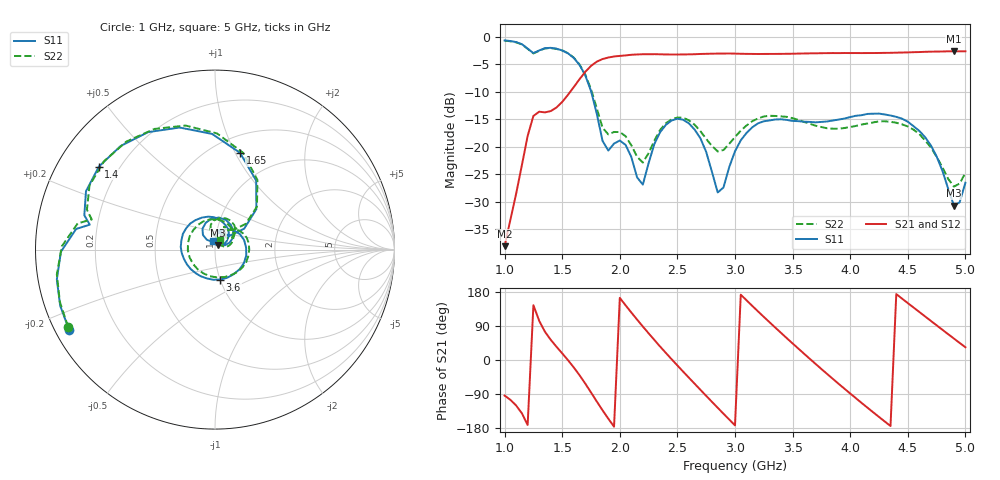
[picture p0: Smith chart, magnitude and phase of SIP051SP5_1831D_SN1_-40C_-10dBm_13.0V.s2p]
# GHz  S  dB  R  50
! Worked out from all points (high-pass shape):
!   81 points, 1 GHz to 5 GHz, reference 50 ohm
!   highest |S21| = -2.62 dB at 4.9 GHz (marker M1); lowest = -38.1 dB at 1 GHz (marker M2)
!   |S21| within 3 dB of the highest: 1.735 GHz to end of sweep
!   lowest |S11| = -30.7 dB at 4.9 GHz (marker M3), VSWR 1.06, Z = 51.7 + j2.44 ohm
!   |S11| at or under -10 dB: 1.752 GHz to end of sweep
!   |S22| runs from -27.2 to -0.7 dB; largest |S21 - S12| = 0.0023
!   S11 on the Smith chart (normalised r, x): 1 GHz: 0.04, -0.26; 1.4 GHz: 0.13, +0.32; 1.65 GHz: 0.67, +1.05; 3.6 GHz: 1.00, -0.34; 5 GHz: 0.97, +0.09
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1  -0.65 -151.2  -38.09 -93.9  -37.92 -92.7  -0.68 -152.2
1.25  -2.96 168.8  -14.39 144.8  -14.38 144.5  -3.01 166.3
1.4  -1.99 144.4  -13.51 53.5  -13.53 53.5  -2.04 141.5
1.55  -3.00 106.2  -10.55 -0.4  -10.56 -0.4  -2.97 103.3
1.65  -5.08 75.5  -7.71 -40.0  -7.70 -40.0  -5.01 73.8
1.7  -6.98 59.2  -6.37 -62.2  -6.37 -62.1  -6.85 58.6
1.85  -18.91 43.2  -4.03 -132.6  -4.02 -132.7  -16.51 46.9
2  -18.86 76.5  -3.46 163.9  -3.44 163.9  -17.32 66.3
2.2  -26.88 108.2  -3.16 88.3  -3.17 88.4  -22.87 83.5
2.35  -17.35 120.9  -3.17 35.5  -3.16 35.5  -16.92 99.2
2.5  -14.89 83.2  -3.21 -14.5  -3.20 -14.5  -14.67 71.2
2.7  -18.47 33.2  -3.11 -78.7  -3.10 -78.7  -17.16 38.1
2.85  -28.31 42.6  -3.04 -126.1  -3.05 -126.1  -20.85 44.5
3  -20.81 80.2  -3.05 -172.5  -3.04 -172.4  -18.23 57.0
3.3  -15.21 4.1  -3.10 99.6  -3.11 99.5  -14.36 10.5
3.6  -15.44 -80.2  -3.02 16.4  -3.02 16.5  -15.49 -57.4
3.7  -15.55 -106.0  -2.99 -10.4  -2.99 -10.4  -16.17 -85.6
4  -14.59 -174.3  -2.94 -88.4  -2.95 -88.4  -16.40 -178.5
4.35  -14.31 112.1  -2.90 -174.3  -2.91 -174.3  -15.46 88.5
4.65  -18.24 51.2  -2.72 115.0  -2.73 114.9  -18.84 28.4
4.9  -30.71 54.0  -2.62 56.7  -2.62 56.6  -27.25 35.4
5  -26.55 105.3  -2.62 33.6  -2.63 33.6  -24.75 64.3
